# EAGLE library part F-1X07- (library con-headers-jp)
FEMALE HEADER
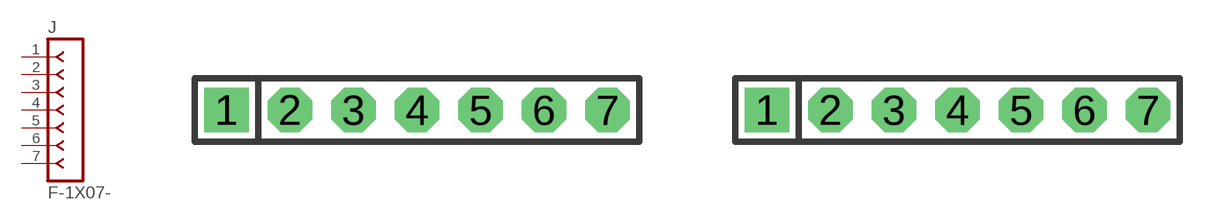
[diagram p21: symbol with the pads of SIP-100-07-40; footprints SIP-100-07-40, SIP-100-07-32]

Designator prefix J

## F-1X07-SIP-100-40  [SIP-100-07-40]
1  1  pas
2  2  pas
3  3  pas
4  4  pas
5  5  pas
6  6  pas
7  7  pas

## F-1X07-SIP-100-32  [SIP-100-07-32]
Pads as for SIP-100-07-40

## F-1X07-SIP-100-32Y  [SIP-100-07-32Y]
Pads as for SIP-100-07-40

## F-1X07-SIP-100-40Y  [SIP-100-07-40Y]
Pads as for SIP-100-07-40

## Footprint SIP-100-07-40 (pad centres in mm)
SIP Header - 0.1", 40 mil drill
drill 1.016 pad 1.778 square: 1 -7.62,0
drill 1.016 pad 1.778 octagon: 2 -5.08,0; 3 -2.54,0; 4 0,0; 5 2.54,0; 6 5.08,0; 7 7.62,0

## Footprint SIP-100-07-32 (pad centres in mm)
SIP Header - 0.1", 32 mil drill
drill 0.813 pad 1.778 square: 1 -7.62,0
drill 0.813 pad 1.778 octagon: 2 -5.08,0; 3 -2.54,0; 4 0,0; 5 2.54,0; 6 5.08,0; 7 7.62,0

## Footprint SIP-100-07-32Y (pad centres in mm)
SIP Header - 0.1", 32 mil drill
drill 0.813 long: 1 -7.62,0; 2 -5.08,0; 3 -2.54,0; 4 0,0; 5 2.54,0; 6 5.08,0; 7 7.62,0

## Footprint SIP-100-07-40Y (pad centres in mm)
SIP Header - 0.1", 40 mil drill
drill 1.016 long: 1 -7.62,0; 2 -5.08,0; 3 -2.54,0; 4 0,0; 5 2.54,0; 6 5.08,0; 7 7.62,0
